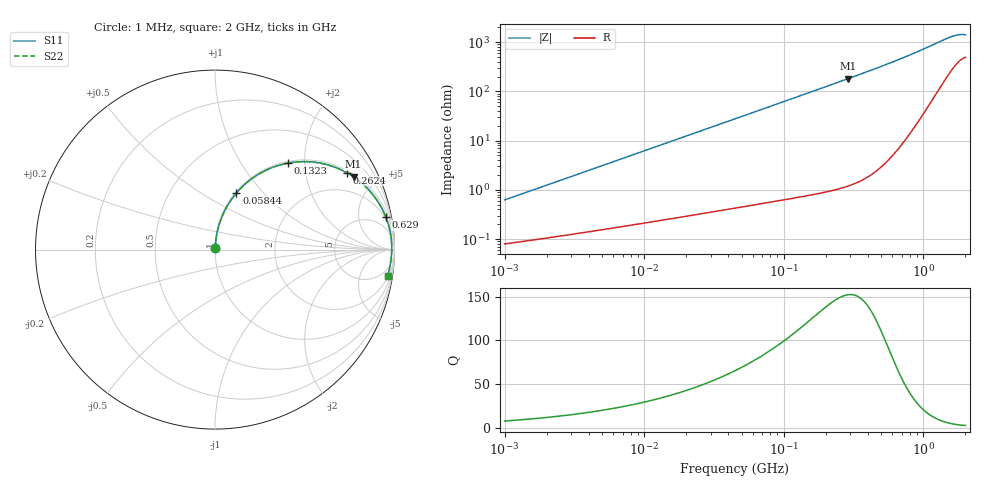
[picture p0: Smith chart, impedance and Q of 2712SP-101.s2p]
# MHz  S  MA  R  50
!Freq  MagS11  AngS11  MagS21  AngS21  MagS12  AngS12  MagS22  AngS22
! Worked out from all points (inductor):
!   801 points, 1 MHz to 2 GHz, reference 50 ohm
!   read as one part in series: L = 98.6 nH near 1.039 MHz
!   highest Q = 152 at 288.5 MHz (marker M1), where L = 100 nH
!   S11 on the Smith chart (normalised r, x): 1 MHz: 1.00, +0.01; 58.44 MHz: 1.01, +0.72; 132.3 MHz: 1.03, +1.65; 262.4 MHz: 1.09, +3.37; 629 MHz: 2, +10; 2 GHz: 2, -13
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1  0.006203 82.3  0.9992 -0.4  0.9992 -0.4  0.006203 82.3
3.573795  0.02201 85.2  0.9984 -1.3  0.9984 -1.3  0.02201 85.2
7.152559  0.04395 85.1  0.9972 -2.5  0.9972 -2.5  0.04395 85.1
12.65119  0.07752 83.8  0.9947 -4.5  0.9947 -4.5  0.07751 83.8
24.6082  0.1494 80.1  0.9856 -8.7  0.9856 -8.7  0.1494 80.1
44.78507  0.2649 73.6  0.9602 -15.5  0.9602 -15.5  0.2649 73.6
58.44032  0.3373 69.3  0.9369 -20.0  0.9369 -20.0  0.3373 69.3
71.35051  0.4008 65.4  0.9114 -23.9  0.9114 -23.9  0.4007 65.4
87.11272  0.471 60.9  0.877 -28.5  0.877 -28.5  0.471 60.9
106.357  0.5462 55.9  0.8324 -33.5  0.8324 -33.5  0.5461 55.9
132.3446  0.6302 49.9  0.771 -39.6  0.771 -39.6  0.6301 49.9
160.0527  0.7007 44.4  0.7079 -45.2  0.7079 -45.2  0.7006 44.4
202.9826  0.7803 37.5  0.6199 -52.1  0.6199 -52.1  0.7801 37.5
262.3676  0.8506 30.2  0.5204 -59.4  0.5204 -59.4  0.8504 30.2
288.5284  0.872 27.7  0.4839 -61.9  0.4839 -61.9  0.8718 27.7
398.5978  0.9274 19.9  0.3678 -69.7  0.3678 -69.7  0.9271 19.9
566.5845  0.9624 12.7  0.2614 -76.6  0.2614 -76.6  0.9621 12.7
629.0293  0.9691 10.8  0.2343 -78.4  0.2343 -78.4  0.9688 10.8
973.9826  0.9838 3.7  0.1411 -83.7  0.1411 -83.7  0.9835 3.7
1566.545  0.9816 -3.8  0.0769 -82.3  0.0769 -82.3  0.9816 -3.8
1789.503  0.9777 -6.3  0.06891 -79.7  0.06891 -79.7  0.9779 -6.3
2000  0.9731 -8.7  0.06854 -78.2  0.06854 -78.2  0.9735 -8.7
